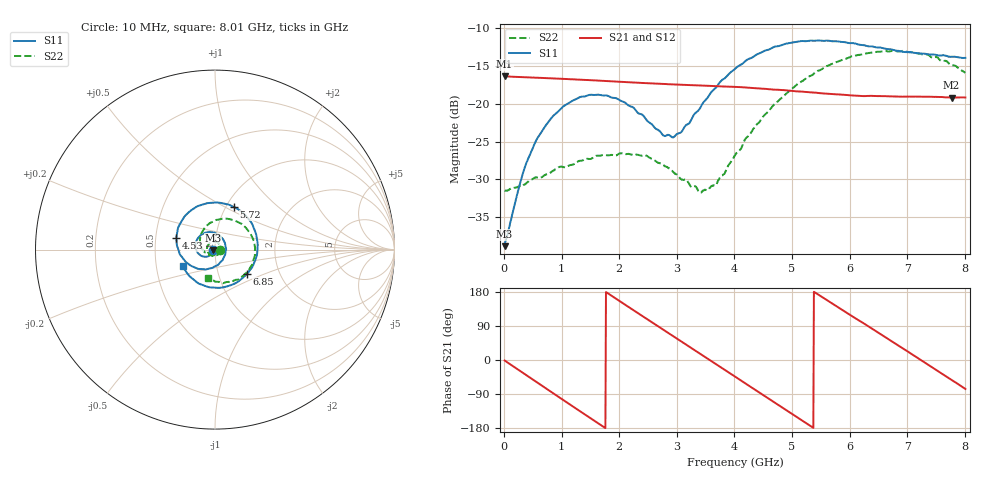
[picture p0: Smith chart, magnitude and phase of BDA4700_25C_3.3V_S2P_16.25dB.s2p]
!Agilent Technologies,E5071B,MY42404982,A.09.10
!Date: Mon Oct 20 18:09:51 2025
!Data & Calibration Information:
!Freq	S11:SOLT2(ON)	S21:SOLT2(ON)	S12:SOLT2(ON)	S22:SOLT2(ON)
# Hz S RI R 50
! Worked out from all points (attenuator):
!   801 points, 10 MHz to 8.01 GHz, reference 50 ohm
!   highest |S21| = -16.34 dB at 10 MHz (marker M1); lowest = -19.2 dB at 7.77 GHz (marker M2)
!   lowest |S11| = -38.9 dB at 10 MHz (marker M3), VSWR 1.02, Z = 48.9 - j0.162 ohm
!   |S11| at or under -10 dB: start of sweep to end of sweep
!   |S22| runs from -31.8 to -13.0 dB; largest |S21 - S12| = 0.0018
!   S11 on the Smith chart (normalised r, x): 10 MHz: 0.98, -0.00; 4.53 GHz: 0.64, +0.09; 5.72 GHz: 1.09, +0.55; 6.85 GHz: 1.37, -0.39; 8.01 GHz: 0.69, -0.13
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1e7  -0.0113 -0.00166  0.1524 -0.00329  0.1523 -0.00341  0.0266 -0.00084
3.3e8  -0.0223 -0.0269  0.124 -0.0848  0.124 -0.0849  0.0233 -0.017
5.6e8  -0.0422 -0.0389  0.0792 -0.1262  0.0791 -0.1262  0.0151 -0.0288
8.7e8  -0.0769 -0.0345  0.00111 -0.1472  0.00127 -0.1472  -0.00704 -0.0358
1.35e9  -0.1097 0.0202  -0.1078 -0.0961  -0.1078 -0.0962  -0.0384 -0.0171
1.96e9  -0.0528 0.0946  -0.132 0.0476  -0.1322 0.0476  -0.034 0.0307
2.45e9  0.0292 0.075  -0.0497 0.1277  -0.0497 0.1279  0.00154 0.0457
2.68e9  0.055 0.0382  0.00379 0.136  0.00358 0.1359  0.0179 0.0365
2.96e9  0.0577 -0.019  0.0657 0.1171  0.0657 0.1169  0.0293 0.0188
3.42e9  -0.0055 -0.0961  0.1277 0.0344  0.1278 0.0344  0.0192 -0.0173
3.67e9  -0.065 -0.1092  0.1291 -0.0222  0.1292 -0.0226  0.000248 -0.0288
4.01e9  -0.152 -0.077  0.0936 -0.0895  0.0937 -0.0893  -0.0362 -0.0276
4.53e9  -0.2154 0.0654  -0.0124 -0.125  -0.0122 -0.1253  -0.0808 0.0263
4.92e9  -0.1665 0.1882  -0.0859 -0.0875  -0.0856 -0.088  -0.0745 0.0926
5.35e9  -0.0311 0.26  -0.1187 -0.00621  -0.1188 -0.00691  -0.0135 0.1544
5.72e9  0.1059 0.2372  -0.0971 0.0634  -0.0971 0.0634  0.072 0.1712
6.23e9  0.2273 0.0905  -0.0158 0.1115  -0.0142 0.1116  0.1847 0.1055
6.68e9  0.2159 -0.0795  0.0657 0.0908  0.066 0.0907  0.2218 -0.0104
6.85e9  0.1793 -0.1345  0.0882 0.0683  0.0886 0.0676  0.2145 -0.058
7.31e9  0.0267 -0.2129  0.1106 -0.0142  0.1108 -0.0143  0.1386 -0.1603
7.77e9  -0.1314 -0.1574  0.0669 -0.0874  0.0668 -0.0875  0.0172 -0.1797
8.01e9  -0.1799 -0.091  0.0258 -0.1071  0.0261 -0.1072  -0.039 -0.1556
